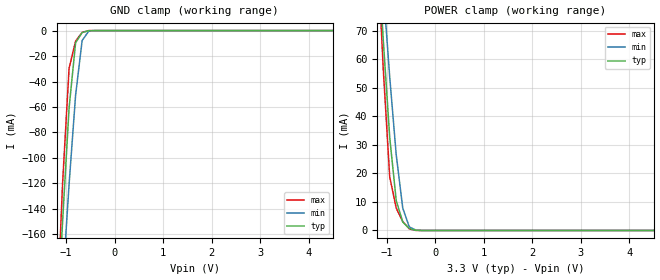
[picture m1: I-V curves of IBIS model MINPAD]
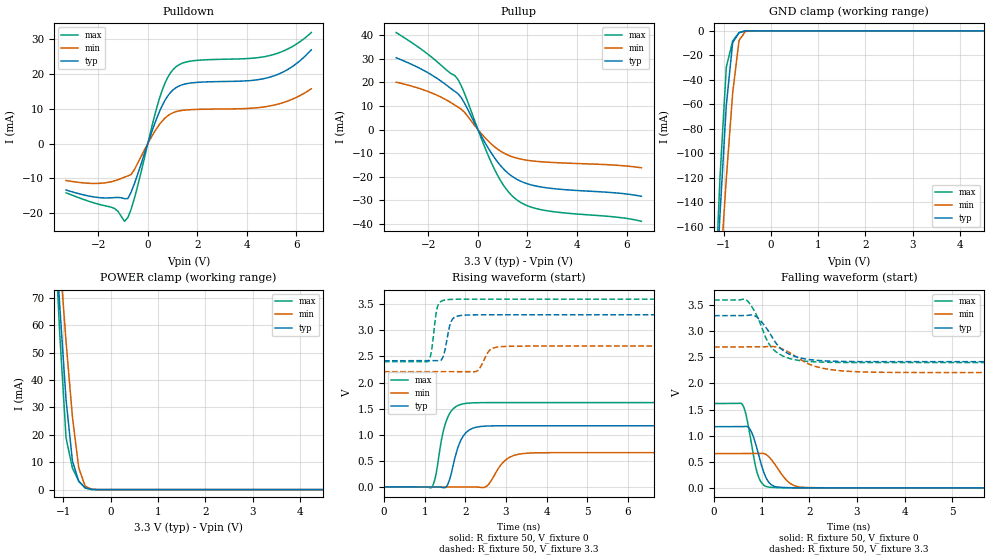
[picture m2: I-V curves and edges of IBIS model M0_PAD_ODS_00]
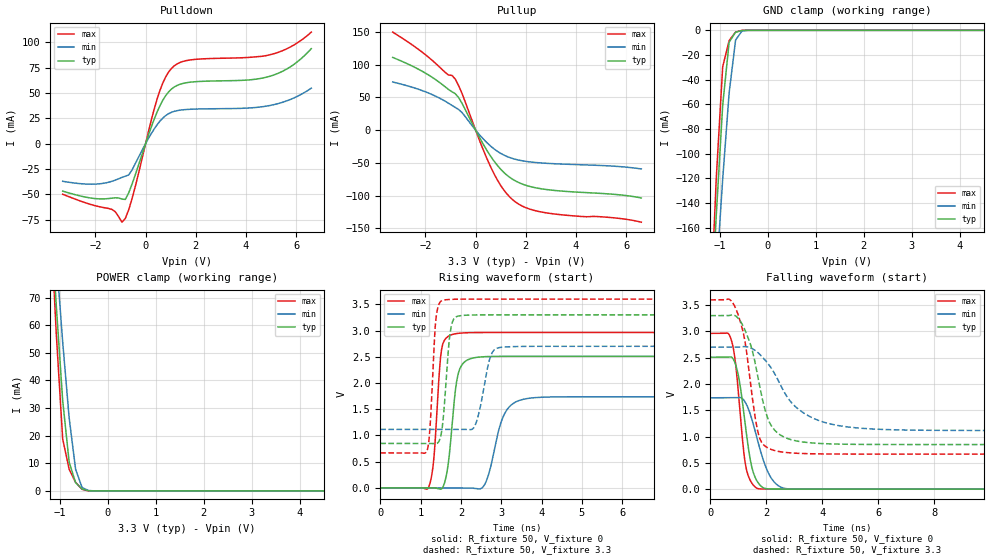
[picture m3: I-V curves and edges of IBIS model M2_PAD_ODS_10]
| Created by SiliconSmart  S-2021.06-SP5-2
[IBIS Ver]   4.0
[File Name]   as320ck_33v_rev1p0.ibs
[File Rev]   1.0
[Date]   Tue Aug 20 2024
|[Source]   Avalanche Team
|[Notes]   Generated IBIS models from Silicon Smart
|[Rev 1.0]   Initial release based on extracted netlist
|[Disclaimer]   THE MODEL LIBRARIES ARE PROVIDED AS IS.
|[Copyright]   Copyright 2024, Avalanche Technology, All Rights Reserved
[Component]   AS30XX20X_BGA
[Manufacturer]  Avalanche Technology
| CONTENT :
| This file contains IBIS MODEL for PSRAM device
| AS30XX20X
| USAGE :
| The models are derived for the 2.7V to 3.6V I/O Operation.
| Temperatures for model generation: typ: 25, max: -40, min: 125
| Voltages : typ: 3.3V, min: 2.7V, max: 3.6V
| PACKAGES SUPPORTED :
| 56-ball FBGA (10mm x 10mm)
| VERIFICATION
| Errors  : 0
| Warnings: 11
| All warnings due to non-monotonic data:
[Package]
|  Design die-package: BGA
| variable   typ   min   max
R_pkg   0.72029   0.51528   1.0002
L_pkg   5.797e-9   4.155e-9   8.073e-9
C_pkg   1.116e-12   7.907e-13   1.753e-12
|Pin and Model info
[Pin]  signal_name  model_name   R_pin   L_pin   C_pin
E2   CS1#   MINPAD   0.4340	15.2000E-9	1.2600E-12
C3   CS2#   MINPAD   0.3800	13.5000E-9	1.0400E-12
D2   CLK1   MINPAD   0.4300	12.7000E-9	0.9790E-12
D1   CLK2   MINPAD   0.4480	14.6000E-9	1.1600E-12
F3   IO_0   MIOPAD   0.4010	12.4000E-9	1.2500E-12
F2   IO_1   MIOPAD   0.4050	14.2000E-9	1.1100E-12
E4   IO_2   MIOPAD   0.3780	11.8000E-9	1.2000E-12
F4   IO_3   MIOPAD   0.3700	11.8000E-9	1.2600E-12
F5   IO_4   MIOPAD   0.3710	11.1000E-9	1.1000E-12
G3   IO_5   MIOPAD   0.4050	13.8000E-9	1.1600E-12
G2   IO_6   MIOPAD   0.3830	15.2000E-9	1.0900E-12
G1   IO_7   MIOPAD   0.4480	16.4000E-9	1.0800E-12
C7   HTBSEL   MINPAD   0.1380	6.1700E-9	0.6060E-12
B7   HBP_2   MINPAD   0.1470	6.3900E-9	1.0000E-12
A6   HBP_1   MINPAD   0.1910	8.5000E-9	1.1500E-12
A5   HBP_0   MINPAD   0.2050	8.6800E-9	1.4200E-12
C4   RESET#   MINPAD   0.3410	14.1000E-9	1.6300E-12
C5   INT1#   MIOPAD   0.3080	12.5000E-9	1.2100E-12
D3   INT2#   MIOPAD   0.2120	10.3000E-9	0.8230E-12
B1   VSSIO   GND   NA   NA   NA
B5   VSSIO   GND   NA   NA   NA
B6   VSSIO   GND   NA   NA   NA
E1   VSSIO   GND   NA   NA   NA
G5   VSSIO   GND   NA   NA   NA
G6   VSSIO   GND   NA   NA   NA
A1   VSS   GND   NA   NA   NA
A3   VSS   GND   NA   NA   NA
B3   VSS   GND   NA   NA   NA
E5   VSS   GND   NA   NA   NA
E6   VSS   GND   NA   NA   NA
E7   VSS   GND   NA   NA   NA
G7   VSS   GND   NA   NA   NA
A8   VSS   GND   NA   NA   NA
A7   VCCIO   POWER   NA   NA   NA
B2   VCCIO   POWER   NA   NA   NA
B4   VCCIO   POWER   NA   NA   NA
C6   VCCIO   POWER   NA   NA   NA
F1   VCCIO   POWER   NA   NA   NA
F6   VCCIO   POWER   NA   NA   NA
G4   VCCIO   POWER   NA   NA   NA
A2   VCC   POWER   NA   NA   NA
A4   VCC   POWER   NA   NA   NA
D4   VCC   POWER   NA   NA   NA
D6   VCC   POWER   NA   NA   NA
D7   VCC   POWER   NA   NA   NA
F7   VCC   POWER   NA   NA   NA
| IOPAD
[Model Selector] MIOPAD
| Model Description
M0_PAD_ODS_00   35ohms
M1_PAD_ODS_01   40ohms
M2_PAD_ODS_10   20ohms
M3_PAD_ODS_11   15ohms
| Models and submodels in the file (5): MINPAD (Input), M0_PAD_ODS_00 (I/O), M2_PAD_ODS_10 (I/O), M1_PAD_ODS_01 (I/O), M3_PAD_ODS_11 (I/O)
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[Model] MINPAD
Model_type Input
Enable   Active-High
Vinl  =  0.8
Vinh  =  2.2
| Capacitance  typ   min   max
C_comp   1.514972e-12   1.421422e-12   1.647034e-12
| Variables   typ   min   max
[GND Clamp Reference]   0   0   0
[POWER Clamp Reference]   3.3   2.7   3.6
[Pulldown Reference]   0   0   0
[Pullup Reference]   3.3   2.7   3.6
[Temperature Range]   25   125   -40
[Voltage Range]   3.3   2.7   3.6
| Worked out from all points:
|   GND clamp passes 1 mA (typ) near -0.62 V on its own axis
|   POWER clamp passes 1 mA (typ) near -0.56 V on its own axis
[GND Clamp]
| Voltage   I(typ)   I(min)   I(max)
-3.3V     -1.961A    -1.697A    -2.357A
-1.21V    -250.6mA   -283.7mA   -242.3mA
-1.076V   -150.5mA   -200.1mA   -120.5mA
-941.4mV  -60.74mA   -120.8mA   -29.57mA
-806.9mV  -9.575mA   -50.7mA    -8.295mA
-672.4mV  -1.554mA   -7.862mA   -1.402mA
-537.9mV  -68.53uA   -503.1uA   -16.84uA
-403.4mV  -562.7nA   -18.5uA    -33.29nA
6.6V      0A         0A         0A
[POWER Clamp]
| Voltage   I(typ)   I(min)   I(max)
-3.3V     772.3mA    673.3mA    930.5mA
-1.21V    105.9mA    117.6mA    104.6mA
-1.076V   67.34mA    85.06mA    57.16mA
-941.4mV  32.71mA    53.93mA    18.82mA
-806.9mV  10.48mA    26.53mA    7.848mA
-672.4mV  2.975mA    7.856mA    3.108mA
-537.9mV  710.9uA    1.248mA    573.1uA
-403.4mV  60.69uA    160.8uA    9.187uA
-269mV    142.4nA    6.118uA    23.26nA
6.6V      0A         0A         0A
[Model] M0_PAD_ODS_00
Model_type I/O
Enable   Active-High
Vinl  =  0.8
Vinh  =  2.2
Vmeas =  1.65
Cref  =  30e-12
| Capacitance  typ   min   max
C_comp   1.518728e-12   1.426995e-12   1.652439e-12
| Variables   typ   min   max
[GND Clamp Reference]   0   0   0
[POWER Clamp Reference]   3.3   2.7   3.6
[Pulldown Reference]   0   0   0
[Pullup Reference]   3.3   2.7   3.6
[Temperature Range]   25   125   -40
[Voltage Range]   3.3   2.7   3.6
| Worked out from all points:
|   slope of the pulldown table from 0 to 0.495 V, typ, clamps not added: 52.1 ohm
|   slope of the pullup table from 0 to 0.495 V, typ, clamps not added: 53.8 ohm
|   GND clamp passes 1 mA (typ) near -0.62 V on its own axis
|   POWER clamp passes 1 mA (typ) near -0.56 V on its own axis
|   falling waveform, R_fixture 50, V_fixture 0: 20-80 % time 230ps typ, 320ps min, 197ps max; typ from 1.17 V to 0 V
|   falling waveform, R_fixture 50, V_fixture 3.3: 20-80 % time 464ps typ, 646ps min, 395ps max; typ from 3.3 V to 2.42 V
|   rising waveform, R_fixture 50, V_fixture 0: 20-80 % time 273ps typ, 362ps min, 248ps max; typ from 0 V to 1.17 V
|   rising waveform, R_fixture 50, V_fixture 3.3: 20-80 % time 138ps typ, 198ps min, 113ps max; typ from 2.42 V to 3.3 V
[GND Clamp]
| Voltage   I(typ)   I(min)   I(max)
-3.3V     -1.961A    -1.697A    -2.357A
-1.21V    -250.6mA   -283.7mA   -242.3mA
-1.076V   -150.5mA   -200.1mA   -120.5mA
-941.4mV  -60.74mA   -120.8mA   -29.57mA
-806.9mV  -9.575mA   -50.7mA    -8.297mA
-672.4mV  -1.554mA   -7.862mA   -1.403mA
-537.9mV  -68.54uA   -503.1uA   -16.86uA
-403.4mV  -562.8nA   -18.5uA    -33.35nA
6.6V      0A         0A         0A
[POWER Clamp]
| Voltage   I(typ)   I(min)   I(max)
-3.3V     772.3mA    673.3mA    930.5mA
-1.21V    105.9mA    117.6mA    104.6mA
-1.076V   67.34mA    85.06mA    57.16mA
-941.4mV  32.71mA    53.93mA    18.82mA
-806.9mV  10.48mA    26.53mA    7.848mA
-672.4mV  2.975mA    7.856mA    3.108mA
-537.9mV  710.9uA    1.248mA    573.1uA
-403.4mV  60.69uA    160.8uA    9.187uA
-269mV    142.4nA    6.118uA    23.26nA
6.6V      0A         0A         0A
[Pulldown]
| Voltage   I(typ)   I(min)   I(max)
-3.3V     -13.3mA    -10.58mA   -14.1mA
-1.345V   -15.45mA   -10.67mA   -18.57mA
-941.4mV  -15.77mA   -9.613mA   -22.25mA
-806.9mV  -15.75mA   -9.264mA   -21.18mA
-537.9mV  -11.42mA   -7.417mA   -15.59mA
455.2mV   8.881mA    5.308mA    12.55mA
682.8mV   12.23mA    7.205mA    17.1mA
1.024V    15.38mA    8.837mA    21.2mA
1.821V    17.39mA    9.724mA    23.68mA
4.914V    18.96mA    10.73mA    25.16mA
5.783V    21.77mA    12.53mA    27.53mA
6.6V      26.8mA     15.66mA    31.75mA
[Pullup]
| Voltage   I(typ)   I(min)   I(max)
-3.3V     30.5mA     20.14mA    41.2mA
-1.883V   23.29mA    15.62mA    30.87mA
-806.9mV  15.25mA    9.542mA    21.3mA
-537.9mV  11.15mA    7.295mA    15.28mA
227.6mV   -4.454mA   -2.797mA   -6.218mA
682.8mV   -12.19mA   -7.423mA   -17.18mA
1.138V    -17.82mA   -10.5mA    -25.22mA
1.593V    -21.27mA   -12.22mA   -30.06mA
2.048V    -23.21mA   -13.14mA   -32.59mA
2.731V    -24.7mA    -13.81mA   -34.4mA
5.659V    -27mA      -15.21mA   -37.28mA
6.6V      -28.37mA   -16.24mA   -38.98mA
[Ramp]
dV/dt_r   0.703466/0.273178n  0.393939/0.362038n  0.969985/0.247584n
dV/dt_f   0.529393/0.464293n  0.294233/0.646299n  0.719381/0.395084n
R_load = 50
[Falling Waveform]
R_fixture = 50
V_fixture = 0
V_fixture_min = 0
V_fixture_max = 0
| Time   V(typ)   V(min)   V(max)
0s        1.172V     656.6mV    1.617V
592.4ps   1.173V     656.8mV    1.6V
665.6ps   1.178V     656.9mV    1.421V
759.8ps   1.115V     656.9mV    978.1mV
915.5ps   703.7mV    658.2mV    254.8mV
1.066ns   243.3mV    651.5mV    35.94mV
1.199ns   60.61mV    545.4mV    10.3mV
1.578ns   3.519mV    98.71mV    1.207mV
1.999ns   806uV      5.289mV    755.6uV
21.88ns   -327.7nV   242.7nV    -127nV
[Falling Waveform]
R_fixture = 50
V_fixture = 3.3
V_fixture_min = 2.7
V_fixture_max = 3.6
| Time   V(typ)   V(min)   V(max)
0s        3.3V       2.7V       3.6V
665.9ps   3.302V     2.701V     3.608V
902.6ps   3.269V     2.701V     3.289V
1.118ns   3.036V     2.709V     2.812V
1.263ns   2.823V     2.707V     2.637V
1.596ns   2.554V     2.586V     2.476V
2.098ns   2.448V     2.337V     2.415V
2.677ns   2.423V     2.243V     2.403V
3.589ns   2.418V     2.213V     2.402V
21.88ns   2.418V     2.21V      2.401V
[Rising Waveform]
R_fixture = 50
V_fixture = 0
V_fixture_min = 0
V_fixture_max = 0
| Time   V(typ)   V(min)   V(max)
0s        11.69nV    88.39nV    -29.68nV
1.171ns   -780.7uV   -409.6uV   -10.52mV
1.261ns   -840.7uV   -441.1uV   173.8mV
1.555ns   28.57mV    -543.7uV   1.311V
1.822ns   761.8mV    -637.1uV   1.56V
2.034ns   1.053V     -711.2uV   1.603V
2.51ns    1.166V     3.888mV    1.616V
3.037ns   1.171V     542.1mV    1.616V
3.713ns   1.172V     652.4mV    1.616V
21.88ns   1.172V     656.6mV    1.617V
[Rising Waveform]
R_fixture = 50
V_fixture = 3.3
V_fixture_min = 2.7
V_fixture_max = 3.6
| Time   V(typ)   V(min)   V(max)
0s        2.418V     2.21V      2.401V
1.086ns   2.419V     2.21V      2.406V
1.162ns   2.419V     2.21V      2.573V
1.322ns   2.419V     2.21V      3.467V
1.456ns   2.502V     2.21V      3.575V
1.582ns   2.967V     2.21V      3.592V
1.809ns   3.275V     2.211V     3.598V
2.277ns   3.299V     2.216V     3.599V
3.095ns   3.3V       2.696V     3.599V
21.88ns   3.3V       2.7V       3.6V
[Model] M2_PAD_ODS_10
Model_type I/O
Enable   Active-High
Vinl  =  0.8
Vinh  =  2.2
Vmeas =  1.65
Cref  =  30e-12
| Capacitance  typ   min   max
C_comp   1.518728e-12   1.426995e-12   1.652439e-12
| Variables   typ   min   max
[GND Clamp Reference]   0   0   0
[POWER Clamp Reference]   3.3   2.7   3.6
[Pulldown Reference]   0   0   0
[Pullup Reference]   3.3   2.7   3.6
[Temperature Range]   25   125   -40
[Voltage Range]   3.3   2.7   3.6
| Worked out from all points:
|   slope of the pulldown table from 0 to 0.495 V, typ, clamps not added: 14.9 ohm
|   slope of the pullup table from 0 to 0.495 V, typ, clamps not added: 14.7 ohm
|   GND clamp passes 1 mA (typ) near -0.62 V on its own axis
|   POWER clamp passes 1 mA (typ) near -0.56 V on its own axis
|   falling waveform, R_fixture 50, V_fixture 0: 20-80 % time 395ps typ, 590ps min, 315ps max; typ from 2.51 V to 0 V
|   falling waveform, R_fixture 50, V_fixture 3.3: 20-80 % time 660ps typ, 1.32ns min, 478ps max; typ from 3.3 V to 0.848 V
|   rising waveform, R_fixture 50, V_fixture 0: 20-80 % time 197ps typ, 348ps min, 149ps max; typ from 0 V to 2.51 V
|   rising waveform, R_fixture 50, V_fixture 3.3: 20-80 % time 146ps typ, 240ps min, 115ps max; typ from 0.848 V to 3.3 V
[GND Clamp]
| Voltage   I(typ)   I(min)   I(max)
-3.3V     -1.961A    -1.697A    -2.357A
-1.21V    -250.6mA   -283.7mA   -242.3mA
-1.076V   -150.5mA   -200.1mA   -120.5mA
-941.4mV  -60.74mA   -120.8mA   -29.57mA
-806.9mV  -9.575mA   -50.7mA    -8.297mA
-672.4mV  -1.554mA   -7.862mA   -1.403mA
-537.9mV  -68.54uA   -503.1uA   -16.86uA
-403.4mV  -562.8nA   -18.5uA    -33.35nA
6.6V      0A         0A         0A
[POWER Clamp]
| Voltage   I(typ)   I(min)   I(max)
-3.3V     772.3mA    673.3mA    930.5mA
-1.21V    105.9mA    117.6mA    104.6mA
-1.076V   67.34mA    85.06mA    57.16mA
-941.4mV  32.71mA    53.93mA    18.82mA
-806.9mV  10.48mA    26.53mA    7.848mA
-672.4mV  2.975mA    7.856mA    3.108mA
-537.9mV  710.9uA    1.248mA    573.1uA
-403.4mV  60.69uA    160.8uA    9.187uA
-269mV    142.4nA    6.118uA    23.26nA
6.6V      0A         0A         0A
[Pulldown]
| Voltage   I(typ)   I(min)   I(max)
-3.3V     -46.87mA   -37.17mA   -49.98mA
-1.345V   -53.85mA   -37.22mA   -64.92mA
-941.4mV  -54.78mA   -33.33mA   -77.57mA
-806.9mV  -55.07mA   -32.17mA   -73.84mA
-537.9mV  -39.91mA   -25.92mA   -54.28mA
455.2mV   31.02mA    18.55mA    43.7mA
682.8mV   42.73mA    25.18mA    59.65mA
1.024V    53.77mA    30.89mA    74.07mA
1.821V    60.81mA    33.99mA    82.81mA
4.914V    66.31mA    37.51mA    87.55mA
5.783V    76.16mA    43.8mA     95.68mA
6.6V      93.82mA    54.81mA    110.2mA
[Pullup]
| Voltage   I(typ)   I(min)   I(max)
-3.3V     111mA      73.41mA    149.7mA
-1.883V   84.38mA    56.73mA    111.6mA
-806.9mV  55.53mA    34.57mA    77.79mA
-537.9mV  40.76mA    26.67mA    55.77mA
227.6mV   -16.28mA   -10.22mA   -22.7mA
682.8mV   -44.55mA   -27.13mA   -62.75mA
1.138V    -65.13mA   -38.37mA   -92.17mA
1.593V    -77.74mA   -44.67mA   -109.9mA
2.162V    -86.08mA   -48.57mA   -120.7mA
2.845V    -90.86mA   -50.76mA   -126.6mA
5.534V    -98.17mA   -55.18mA   -134.1mA
6.6V      -103.7mA   -59.31mA   -140.6mA
[Ramp]
dV/dt_r   1.5056/0.196832n  1.04252/0.347593n  1.77761/0.148643n
dV/dt_f   1.47118/0.659579n  0.951014/1.31696n  1.76015/0.477784n
R_load = 50
[Falling Waveform]
R_fixture = 50
V_fixture = 0
V_fixture_min = 0
V_fixture_max = 0
| Time   V(typ)   V(min)   V(max)
0s        2.509V     1.738V     2.963V
748.3ps   2.513V     1.738V     2.844V
872ps     2.419V     1.738V     2.517V
989.9ps   2.199V     1.741V     1.925V
1.266ns   1.159V     1.638V     439.8mV
1.472ns   445mV      1.353V     123.4mV
1.698ns   130.7mV    910.7mV    10.93mV
2.175ns   3.503mV    211mV      1.352mV
2.759ns   1.04mV     7.271mV    450uV
21.88ns   562.7nV    40.89nV    -434.7nV
[Falling Waveform]
R_fixture = 50
V_fixture = 3.3
V_fixture_min = 2.7
V_fixture_max = 3.6
| Time   V(typ)   V(min)   V(max)
0s        3.3V       2.7V       3.6V
666.9ps   3.3V       2.701V     3.613V
930.5ps   3.284V     2.701V     3.411V
1.224ns   3.044V     2.711V     2.855V
1.734ns   2.04V      2.581V     1.021V
2.011ns   1.41V      2.421V     798.4mV
2.346ns   1.097V     2.153V     727.6mV
3.37ns    892.8mV    1.437V     676.2mV
5.289ns   851.5mV    1.162V     666.9mV
21.88ns   848mV      1.115V     666.4mV
[Rising Waveform]
R_fixture = 50
V_fixture = 0
V_fixture_min = 0
V_fixture_max = 0
| Time   V(typ)   V(min)   V(max)
0s        5.58nV     44.82nV    -6.256nV
1.197ns   853.2uV    -370.5uV   8.516mV
1.321ns   941.8uV    -409uV     503.5mV
1.529ns   -11.73mV   -473.2uV   2.676V
1.684ns   449.8mV    -521.2uV   2.889V
1.875ns   1.932V     -580.4uV   2.941V
2.554ns   2.501V     25.35mV    2.962V
3.082ns   2.509V     1.413V     2.962V
3.686ns   2.509V     1.709V     2.962V
21.88ns   2.509V     1.738V     2.963V
[Rising Waveform]
R_fixture = 50
V_fixture = 3.3
V_fixture_min = 2.7
V_fixture_max = 3.6
| Time   V(typ)   V(min)   V(max)
0s        848mV      1.115V     666.4mV
1.16ns    847.6mV    1.116V     713.2mV
1.379ns   845.2mV    1.116V     3.219V
1.584ns   1.526V     1.116V     3.582V
1.756ns   3.063V     1.116V     3.594V
2.026ns   3.286V     1.116V     3.599V
2.341ns   3.297V     1.177V     3.599V
2.73ns    3.299V     2.496V     3.599V
3.013ns   3.299V     2.682V     3.599V
21.88ns   3.3V       2.7V       3.6V
